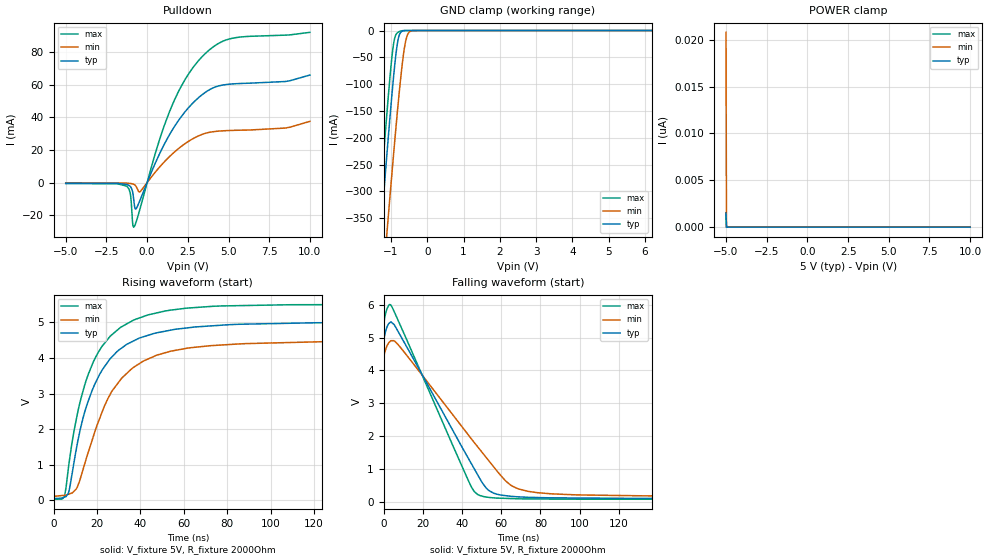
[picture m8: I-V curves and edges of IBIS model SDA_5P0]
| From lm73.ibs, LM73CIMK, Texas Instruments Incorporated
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|   Model SDA_5P0
[Model]   SDA_5P0
Model_type   I/O_open_drain
Polarity   Non-Inverting
Enable   Active-Low
Vinl = 1.5
Vinh = 3.5
Vmeas = 2.5
Vref = 5
Cref = 1pF
Rref = 2000
|   typ   min   max
|   (nom PVT)   (fast PVT)   (slow PVT)
C_comp   0.602p   0.543p   0.661p
|C_comp (ON state)   0.749p   0.730p   0.751p
|C_comp (OFF state)   0.618p   0.558p   0.677p
[Model spec]
|subparameter
Vinl   1.5   1.35   1.65
Vinh   3.5   3.15   3.85
[Voltage Range]   5   4.5   5.5
[Temperature Range]   27   150   -40
[Pullup Reference]   5   4.5   5.5
[Pulldown Reference]   0   -0   0
[Power Clamp Reference]   5   4.5   5.5
[GND Clamp Reference]   0   0   0
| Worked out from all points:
|   slope of the pulldown table from 0 to 0.75 V, typ, clamps not added: 43.3 ohm
|   GND clamp passes 1 mA (typ) near -0.68 V on its own axis
|   falling waveform, V_fixture 5V, R_fixture 2000Ohm: 20-80 % time 27.3ns typ, 34ns min, 23.8ns max; typ from 5 V to 0.097 V
|   rising waveform, V_fixture 5V, R_fixture 2000Ohm: 20-80 % time 17.3ns typ, 20.4ns min, 16.1ns max; typ from 0.097 V to 5 V
[Pulldown]
|   Voltage   I(typ)   I(min)   I(max)
-5V       -394uA     -141.8uA   -589.2uA
-1.25V    -1.146mA   -337.8uA   -2.191mA
-1.025V   -2.468mA   -540.4uA   -7.282mA
-890mV    -5.806mA   -809.7uA   -24.77mA
-815mV    -11.12mA   -1.087mA   -27.22mA
-665mV    -15.89mA   -2.514mA   -23.81mA
-425mV    -10.48mA   -5.486mA   -15.58mA
1.315V    28.32mA    15.36mA    41.94mA
2.32V     43.27mA    23.8mA     62.97mA
3.25V     52.8mA     29.03mA    75.76mA
5.05V     60.29mA    31.92mA    88mA
10V       65.91mA    37.54mA    92.06mA
[GND Clamp]
|   Voltage   I(typ)   I(min)   I(max)
-5V       -3.718A    -3.697A    -3.742A
-1.355V   -440.9mA   -580.8mA   -368mA
-1.25V    -349.5mA   -492.9mA   -274.4mA
-1.13V    -247.1mA   -393.7mA   -170.7mA
-1.07V    -197.3mA   -344.8mA   -121.2mA
-920mV    -81.55mA   -225.7mA   -22.16mA
-830mV    -28mA      -157.8mA   -4.714mA
-755mV    -6.125mA   -105mA     -1.504mA
-665mV    -676uA     -50.31mA   -221.1uA
-590mV    -96.15uA   -18.65mA   -27.76uA
-410mV    -415.2nA   -365.2uA   -14.59nA
10V       0A         0A         0A
[POWER Clamp]
|   Voltage   I(typ)   I(min)   I(max)
-5V       1.475nA    20.78nA    1.533nA
-4.97V    0A         0A         0A
-4.955V   0A         0A         0A
10V       0A         0A         0A
[Ramp]
R_load = 2000
|   typ   min   max
dV/dt_r   2.94181/1.72887e-08   2.59813/2.02697e-08   3.25788/1.5969e-08
dV/dt_f   2.94174/2.72053e-08   2.60093/3.39522e-08   3.25779/2.37736e-08
[Falling Waveform]
V_fixture = 5V
V_fixture_min = 4.5V
V_fixture_max = 5.5V
R_fixture = 2000Ohm
C_fixture = 0F
|   Time   V(typ)   V(min)   V(max)
0s        5V         4.5V       5.5V
2.708ns   5.436V     4.853V     5.997V
4.318ns   5.454V     4.91V      5.931V
10.46ns   4.861V     4.563V     5.115V
43.41ns   1.302V     2.021V     618.9mV
48.28ns   787.1mV    1.651V     210.2mV
56.08ns   262.1mV    1.068V     115.6mV
64.7ns    164.2mV    510.8mV    94.86mV
73.75ns   133mV      313.6mV    82.48mV
199.9ns   97.09mV    165.1mV    70.34mV
[Rising Waveform]
V_fixture = 5V
V_fixture_min = 4.5V
V_fixture_max = 5.5V
R_fixture = 2000Ohm
C_fixture = 0F
|   Time   V(typ)   V(min)   V(max)
0s        96.53mV    162.6mV    70.16mV
5.101ns   94.83mV    145.8mV    124mV
6.867ns   210.4mV    172.7mV    917.3mV
11.65ns   1.805V     489mV      2.618V
18.19ns   3.148V     1.77V      3.872V
26.69ns   4.015V     3.048V     4.642V
36.86ns   4.478V     3.737V     5.063V
53.96ns   4.781V     4.19V      5.343V
72.18ns   4.898V     4.344V     5.445V
199.9ns   5V         4.493V     5.5V
